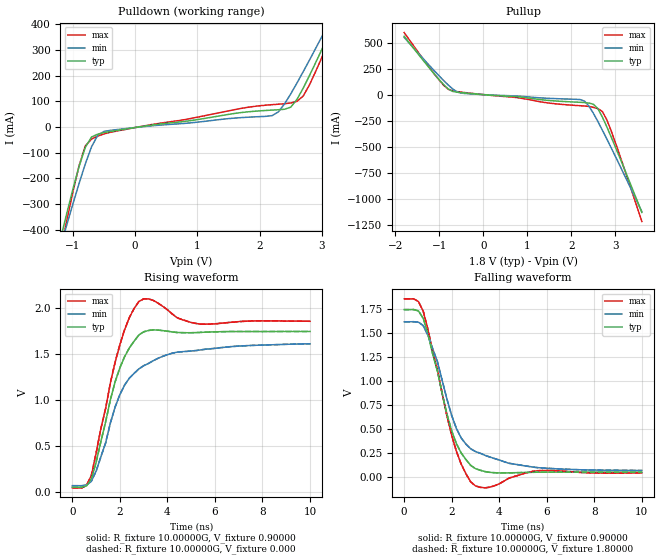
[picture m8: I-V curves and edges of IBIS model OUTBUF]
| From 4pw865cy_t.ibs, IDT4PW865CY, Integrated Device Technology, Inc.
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|   Model OUTBUF
[Model]   OUTBUF
Model_type   Output
Polarity   Inverting
C_comp   6.50000pF   8.10000pF   5.40000pF
[Temperature Range]   25.00000   0.11000k   0.000
[Voltage Range]   1.80000V   1.70000V   1.90000V
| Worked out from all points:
|   slope of the pulldown table from 0 to 0.27 V, typ, clamps not added: 28.1 ohm
|   slope of the pullup table from 0 to 0.27 V, typ, clamps not added: 33.2 ohm
|   rising waveform, R_fixture 10.00000G, V_fixture 0.90000: 20-80 % time 1.03ns typ, 1.46ns min, 898ps max; typ from 0.047 V to 1.74 V
|   rising waveform, R_fixture 10.00000G, V_fixture 0.000: 20-80 % time 1.03ns typ, 1.46ns min, 898ps max; typ from 0.047 V to 1.74 V
|   falling waveform, R_fixture 10.00000G, V_fixture 0.90000: 20-80 % time 1.05ns typ, 1.25ns min, 994ps max; typ from 1.74 V to 0.047 V
|   falling waveform, R_fixture 10.00000G, V_fixture 1.80000: 20-80 % time 1.05ns typ, 1.25ns min, 994ps max; typ from 1.74 V to 0.047 V
[Pulldown]
| voltage   I(typ)   I(min)   I(max)
-1.8V     -1.057A    -989.8mA   -1.241A
-1.2V     -436.7mA   -467mA     -485.7mA
-1.1V     -337.5mA   -382.4mA   -365.9mA
-900mV    -152.9mA   -219.1mA   -149.7mA
-700mV    -38.6mA    -76.63mA   -46.7mA
-500mV    -21.5mA    -16.86mA   -26.51mA
2.2V      66.13mA    44.53mA    87.31mA
2.5V      77.68mA    129.5mA    93.98mA
2.7V      151.9mA    215.9mA    121mA
3.1V      355.4mA    399.3mA    328.7mA
3.2V      408.3mA    446.2mA    386.4mA
3.6V      623.1mA    635.4mA    621.6mA
[Pullup]
| voltage   I(typ)   I(min)   I(max)
-1.8V     560mA      548.9mA    595.6mA
-1.1V     191.5mA    223.1mA    191.6mA
-800mV    56.3mA     93.89mA    53.18mA
-500mV    20.65mA    15.91mA    25.61mA
2.2V      -71.66mA   -45.68mA   -104.4mA
2.3V      -74.07mA   -61.24mA   -106.9mA
2.5V      -90.54mA   -177.7mA   -120.2mA
2.6V      -132.2mA   -254.9mA   -132.5mA
2.7V      -210.6mA   -336.2mA   -158.6mA
2.8V      -302.8mA   -419.8mA   -235.5mA
3V        -501.1mA   -591mA     -459.3mA
3.6V      -1.126A    -1.118A    -1.213A
[Ramp]
| variable   typ   min   max
dV/dt_r   1.01813/0.97004n   0.92698/1.41193n   1.08859/0.84164n
dV/dt_f   1.01814/0.98696n   0.93113/1.19441n   1.08956/0.93599n
R_load = 10.00000G
[Rising Waveform]
R_fixture = 10.00000G
V_fixture = 0.90000
V_fixture_min = 0.85000
V_fixture_max = 0.95000
| time   V(typ)   V(min)   V(max)
0s        47.11mV    64.03mV    40.69mV
600ps     62.29mV    71.17mV    69.66mV
800ps     136.9mV    112.5mV    175.6mV
2ns       1.347V     1.056V     1.599V
2.4ns     1.565V     1.236V     1.895V
2.8ns     1.706V     1.336V     2.07V
3.4ns     1.761V     1.425V     2.083V
4.4ns     1.733V     1.518V     1.895V
5.4ns     1.734V     1.543V     1.824V
10ns      1.744V     1.609V     1.855V
[Rising Waveform]
R_fixture = 10.00000G
V_fixture = 0.000
V_fixture_min = 0.000
V_fixture_max = 0.000
| time   V(typ)   V(min)   V(max)
0s        47.11mV    64.03mV    40.69mV
600ps     62.29mV    71.17mV    69.66mV
800ps     136.9mV    112.5mV    175.6mV
2ns       1.347V     1.056V     1.599V
2.4ns     1.565V     1.236V     1.895V
2.8ns     1.706V     1.336V     2.07V
3.4ns     1.761V     1.425V     2.083V
4.4ns     1.733V     1.518V     1.895V
5.4ns     1.734V     1.543V     1.824V
10ns      1.744V     1.609V     1.855V
[Falling Waveform]
R_fixture = 10.00000G
V_fixture = 0.90000
V_fixture_min = 0.85000
V_fixture_max = 0.95000
| time   V(typ)   V(min)   V(max)
0s        1.744V     1.617V     1.856V
600ps     1.73V      1.613V     1.828V
800ps     1.654V     1.577V     1.728V
1.4ns     1.102V     1.2V       1.116V
2ns       476.2mV    637.7mV    430.4mV
2.4ns     246.9mV    403.6mV    130.5mV
3ns       83.95mV    262.2mV    -96.34mV
3.6ns     45.51mV    205.1mV    -109.9mV
5.6ns     46.6mV     94.33mV    62mV
10ns      47.1mV     65.11mV    40.07mV
[Falling Waveform]
R_fixture = 10.00000G
V_fixture = 1.80000
V_fixture_min = 1.70000
V_fixture_max = 1.90000
| time   V(typ)   V(min)   V(max)
0s        1.744V     1.617V     1.856V
600ps     1.73V      1.613V     1.828V
800ps     1.654V     1.577V     1.728V
1.4ns     1.102V     1.2V       1.116V
2ns       476.2mV    637.7mV    430.4mV
2.4ns     246.9mV    403.6mV    130.5mV
3ns       83.95mV    262.2mV    -96.34mV
3.6ns     45.51mV    205.1mV    -109.9mV
5.6ns     46.6mV     94.33mV    62mV
10ns      47.1mV     65.11mV    40.07mV
